FUNCTION_BLOCK WriteFileOnDisk	//Opens/creates, writes, then closes a file on disk
VAR_INPUT
	Execute : BOOL;	//Execution of the function block begins on a rising edge of this input
	file_path : STRING(255);	//Location of the file on the disk
	file_size : DINT;	//Number of bytes to write to the file 
END_VAR
VAR_OUTPUT
	Done : BOOL;	//Function block is finished, any returned values can be used
END_VAR
VAR_IN_OUT
	data : ARRAY[*] OF SINT;	//data to write to the file as a raw binary
END_VAR
VAR
	file_open : FB_FileOpen;
	file_write : FB_FileWrite;
	file_close : FB_FileClose;
END_VAR


file_open(sNetId := '',sPathName := file_path,nMode := FOPEN_MODEWRITE OR FOPEN_MODEBINARY,ePath := PATH_GENERIC,bExecute := Execute,tTimeout := T#10S);

file_write(sNetId := '',hFile := file_open.hFile,pWriteBuff := data,cbWriteLen := file_size,bExecute := file_open.bExecute AND NOT(file_open.bBusy) AND NOT(file_open.bError),tTimeout := T#10S);

file_close(sNetId := '',hFile := file_open.hFile,bExecute := file_write.bExecute AND NOT(file_write.bBusy) AND NOT(file_write.bError),tTimeout := T#10S);

Done := file_close.bExecute AND NOT(file_close.bBusy) AND NOT(file_close.bError);

END_FUNCTION_BLOCK
